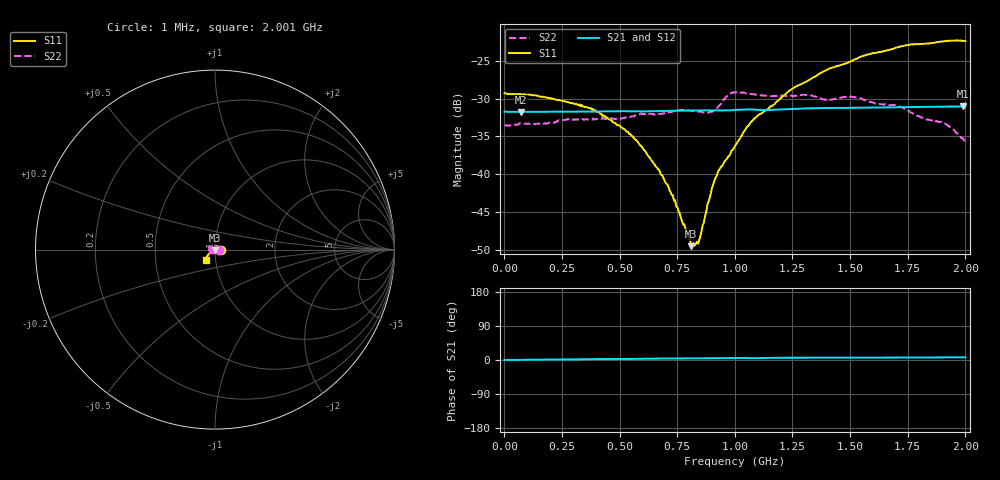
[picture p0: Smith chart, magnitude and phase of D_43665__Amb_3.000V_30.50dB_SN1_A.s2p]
! device id: 43665_
! dir: \\malibu\benchdata\1_engineers\tn_data\43665_75ohm\new\sparar\43665_\amb\3p000v\30p50db
! Serial: 1
! Insertion: A
! Temp: Amb
! VDD: 3.000V
! Attenuation Step: 30.50dB
! IDD: 1.452815e+00mA
! FILE NAME
! DATE 03-27-2009 08:42:05
! CORRECTED  DATA
#  Hz  S  RI  R  75
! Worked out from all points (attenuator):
!   401 points, 1 MHz to 2.001 GHz, reference 75 ohm
!   highest |S21| = -31.05 dB at 1.991 GHz (marker M1); lowest = -31.8 dB at 71 MHz (marker M2)
!   lowest |S11| = -49.5 dB at 811 MHz (marker M3), VSWR 1.01, Z = 75.3 - j0.425 ohm
!   |S11| at or under -10 dB: start of sweep to end of sweep
!   |S22| runs from -35.7 to -29.2 dB; largest |S21 - S12| = 0.00026
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1000000  0.0343 -0.000479  0.0259 2.36e-05  0.0258 -0.000225  0.0212 -0.000133
7.1e7  0.0337 0.000575  0.0258 0.000195  0.0258 0.00021  0.0211 0.00452
3.36e8  0.0285 0.00221  0.0259 0.000866  0.0259 0.000902  0.0127 0.0194
4.11e8  0.0254 0.0029  0.0259 0.00109  0.0259 0.00113  0.00842 0.0216
5.36e8  0.019 0.00199  0.026 0.00129  0.0261 0.00136  0.00146 0.0238
6.71e8  0.0107 -9.4e-05  0.0261 0.00171  0.0261 0.00177  -0.0069 0.024
7.31e8  0.00716 -0.00129  0.0262 0.00186  0.0262 0.00189  -0.0102 0.024
8.11e8  0.00179 -0.00282  0.0263 0.00195  0.0263 0.00203  -0.0155 0.0211
8.21e8  0.00121 -0.00328  0.0263 0.00199  0.0263 0.00204  -0.0161 0.0206
8.41e8  -0.000258 -0.00345  0.0263 0.00204  0.0263 0.0021  -0.0171 0.0195
9.16e8  -0.00633 -0.00696  0.0263 0.00208  0.0263 0.00216  -0.0224 0.0147
9.71e8  -0.00964 -0.00884  0.0263 0.00231  0.0263 0.00237  -0.0299 0.0153
1.001e9  -0.0122 -0.00924  0.0264 0.00244  0.0265 0.00249  -0.0306 0.0164
1.096e9  -0.0199 -0.0135  0.0265 0.00228  0.0266 0.0024  -0.0308 0.0134
1.241e9  -0.0294 -0.0205  0.0268 0.00289  0.0268 0.00299  -0.0322 0.00633
1.336e9  -0.0346 -0.0258  0.0271 0.00292  0.0272 0.00302  -0.033 0.00237
1.406e9  -0.0388 -0.0308  0.0273 0.00283  0.0273 0.00294  -0.0308 -0.00125
1.511e9  -0.0433 -0.0359  0.0273 0.0029  0.0274 0.00301  -0.0321 -0.00439
1.671e9  -0.0483 -0.0454  0.0274 0.00307  0.0275 0.00315  -0.0279 -0.00622
1.906e9  -0.0508 -0.056  0.0277 0.00331  0.0278 0.00341  -0.0207 -0.00667
1.991e9  -0.0494 -0.058  0.0278 0.00344  0.0279 0.00344  -0.0165 -0.00504
2.001e9  -0.0493 -0.0579  0.0278 0.00347  0.0278 0.00344  -0.0159 -0.00435
